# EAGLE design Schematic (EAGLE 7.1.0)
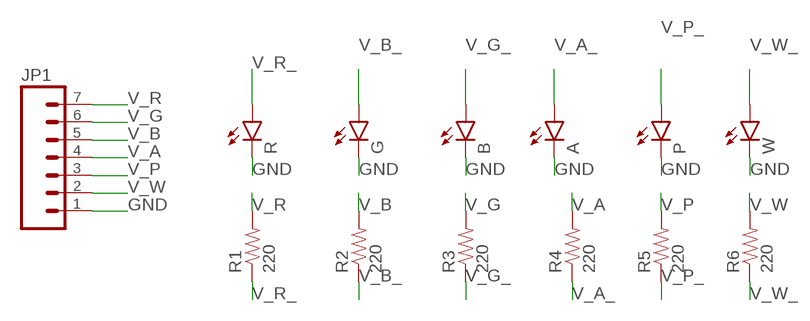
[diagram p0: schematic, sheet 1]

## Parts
A  LED5MM  [LED5MM]
B  LED5MM  [LED5MM]
G  LED5MM  [LED5MM]
JP1  M07  [1X07]
P  LED5MM  [LED5MM]
R  LED5MM  [LED5MM]
R1  220  RESISTOREZ  [AXIAL-0.3EZ]
R2  220  RESISTOREZ  [AXIAL-0.3EZ]
R3  220  RESISTOREZ  [AXIAL-0.3EZ]
R4  220  RESISTOREZ  [AXIAL-0.3EZ]
R5  220  RESISTOREZ  [AXIAL-0.3EZ]
R6  220  RESISTOREZ  [AXIAL-0.3EZ]
W  LED5MM  [LED5MM]

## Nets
GND: A.K(C) B.K(C) G.K(C) JP1.1 P.K(C) R.K(C) W.K(C)
V_A: JP1.4 R4.P$2
V_A_: A.A R4.P$1
V_B: JP1.5 R2.P$2
V_B_: G.A R2.P$1
V_G: JP1.6 R3.P$2
V_G_: B.A R3.P$1
V_P: JP1.3 R5.P$2
V_P_: P.A R5.P$1
V_R: JP1.7 R1.P$2
V_R_: R1.P$1 R.A
V_W: JP1.2 R6.P$2
V_W_: R6.P$1 W.A

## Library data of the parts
A B G P R W = SparkFun-LED:LED: LEDs
JP1 = SparkFun-Connectors:M07: Header 7 Standard 7-pin 0.1" header. Use with straight break away headers (SKU : PRT-00116), right angle break away headers (PRT-00553), swiss pins (PRT-00743), machine pins (PRT-00117), and female headers (PRT-00115). NOTES ON THE VARIANTS LOCK and LOCK_LONGPADS... This footprint was designed to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
R1-R6 = SparkFun-Passives:RESISTOR: Resistor

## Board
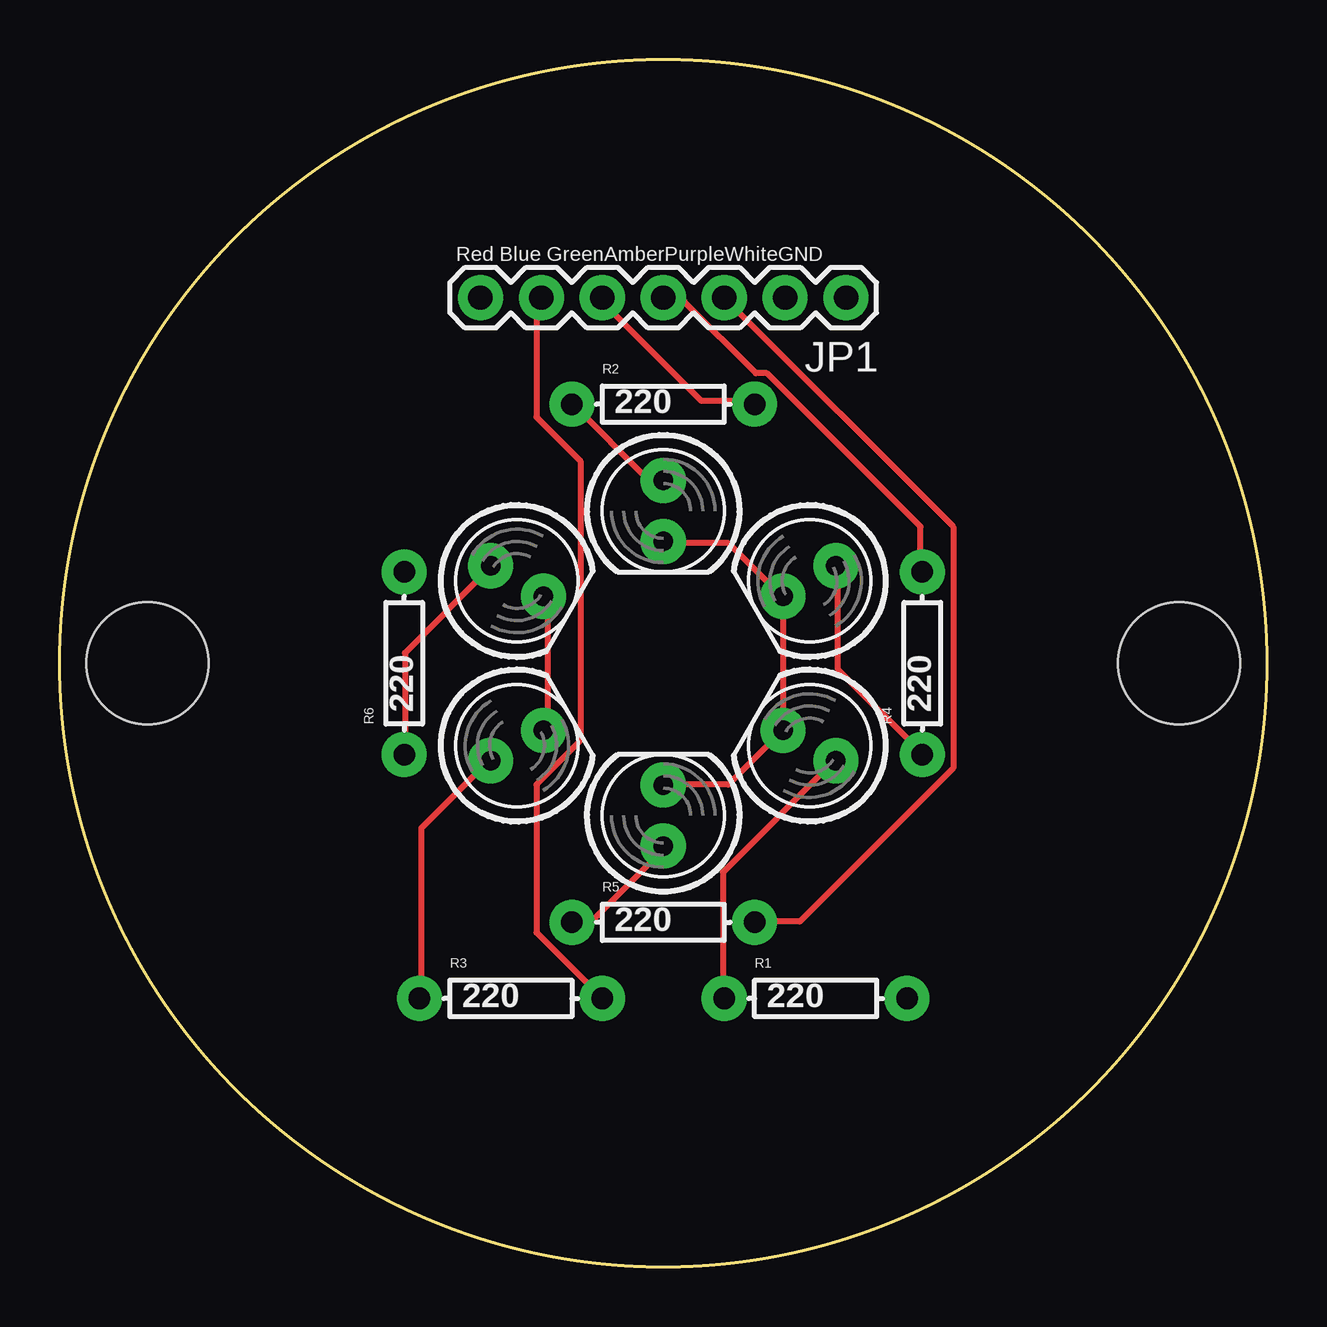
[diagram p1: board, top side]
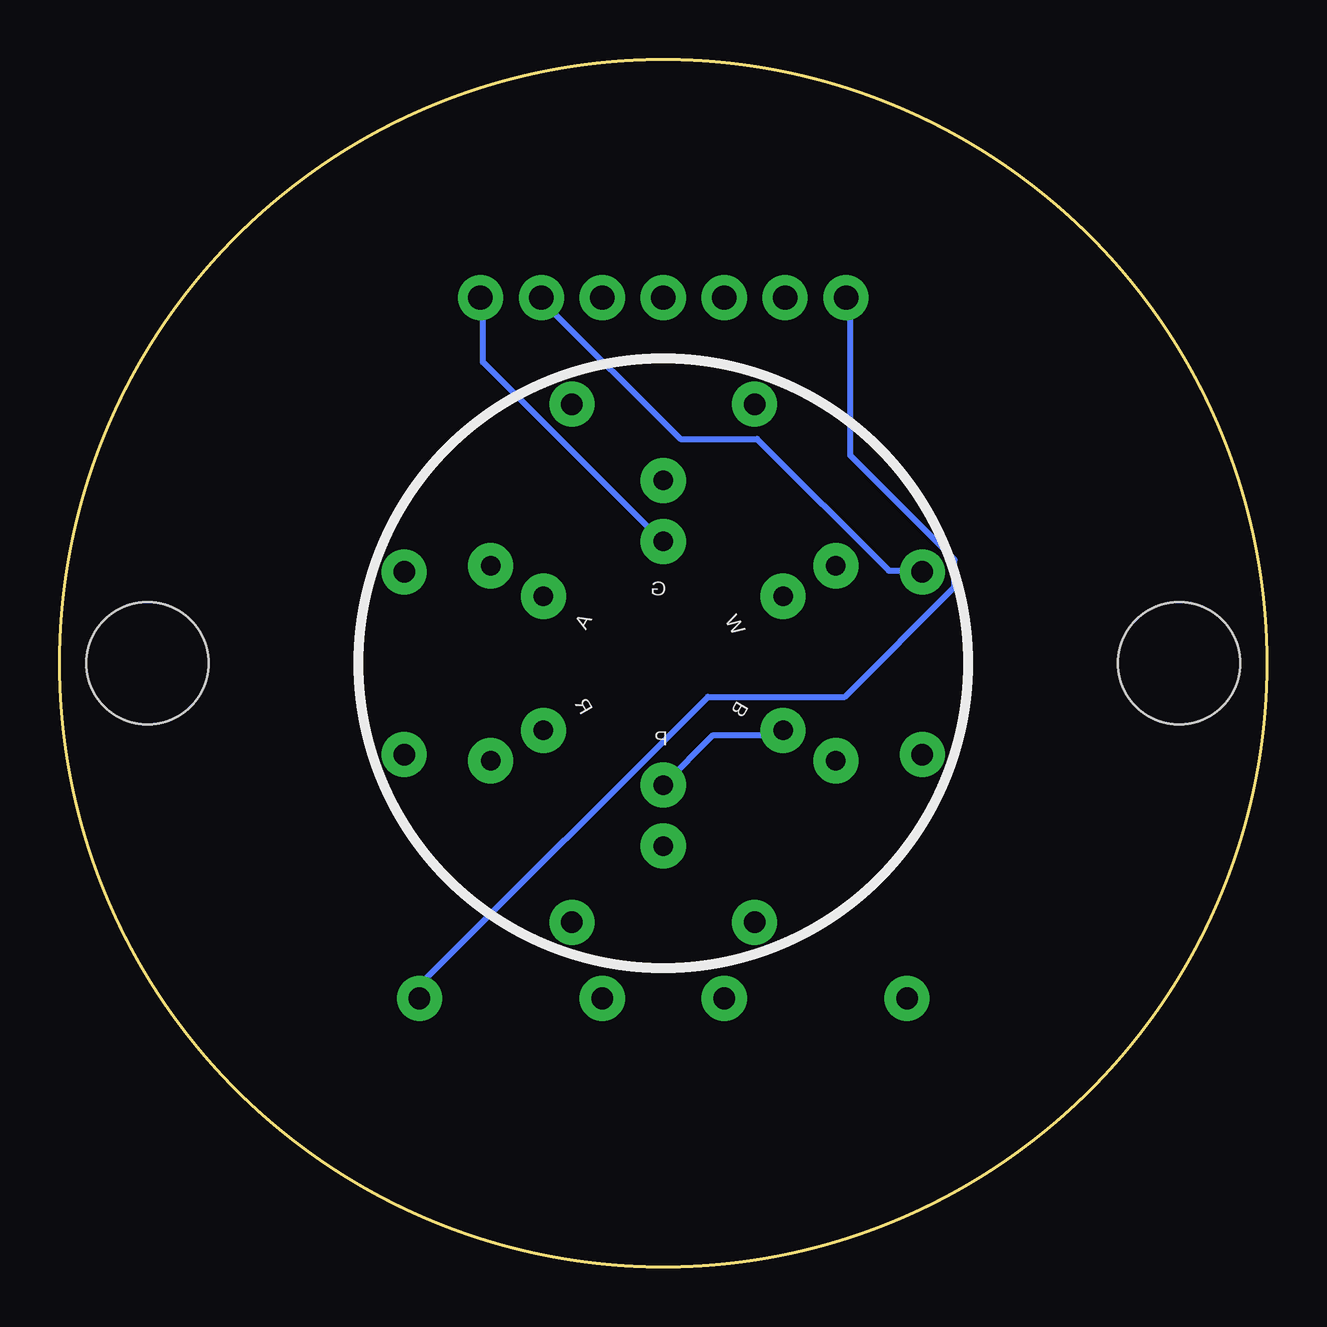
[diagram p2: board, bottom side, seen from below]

Size 50.29 x 50.29 mm. Coordinates in mm from the lower left corner, seen from the top.
Outline: circle at 25.15,25.15 radius 25.15
Copper layers (1*16): Top 0.035mm / dielectric 1.5mm / Bottom 0.035mm
Design rules "default": minimum track width 10mil, minimum drill 24mil, track to track 8mil, track to pad 8mil, pad to pad 8mil, via to via 8mil, smd to smd 8mil, copper to edge 40mil, drill to drill 8mil, minimum pad ring 10mil, minimum via ring 8mil, stop-mask expansion 4mil, vias tented up to drill 0mil, thermal gap 10mil
Holes 5.08 mm at 3.65,25.15 46.65,25.15

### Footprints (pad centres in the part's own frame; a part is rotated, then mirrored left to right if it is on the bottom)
LED5MM = drill 0.813 pad 1.88: A -1.27,0; K 1.27,0
1X07 = drill 1.016 pad 1.88: 1 0,0; 2 2.54,0; 3 5.08,0; 4 7.62,0; 5 10.16,0; 6 12.7,0; 7 15.24,0
AXIAL-0.3EZ = drill 0.9 pad 1.88: P$1 -3.81,0; P$2 3.81,0

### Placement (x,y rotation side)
A  31.24,28.58 210 top
B  19.05,21.72 30 top
G  25.15,31.5 270 top
JP1  32.77,40.39 180 top
P  25.15,18.8 90 top
R  31.24,21.72 150 top
R1  31.5,11.18 0 top
R2  25.15,35.94 0 top
R3  18.8,11.18 0 top
R4  35.94,25.15 90 top
R5  25.15,14.35 0 top
R6  14.35,25.15 90 top
W  19.05,28.58 330 top

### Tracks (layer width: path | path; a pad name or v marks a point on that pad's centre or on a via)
GND
  Top 0.254: B.K 20.32,22.38 20.32,27.86 W.K | P.K 25.35,20.09 27.86,20.09 29.92,22.15 R.K 30.15,22.38 30.15,27.86 A.K 29.92,28.09 27.86,30.15 25.35,30.15 G.K
  Bottom 0.254: JP1.1 32.66,40.21 32.66,37.69 25.35,30.38 G.K | P.K 23.06,22.15 20.32,22.15 B.K
V_A
  Top 0.254: JP1.4 25.35,40.21 26.04,40.21 29.01,37.24 29.46,37.24 35.87,30.84 35.87,29.01 R4.P$2
V_A_
  Top 0.254: A.A 32.44,29.01 32.44,24.89 35.87,21.46 R4.P$1
V_B
  Top 0.254: R2.P$2 28.78,36.09 26.72,36.09 22.61,40.21 JP1.5
V_B_
  Top 0.254: G.A 25.12,32.89 24.44,32.89 21.46,35.87 R2.P$1
V_G
  Top 0.254: R3.P$2 19.86,13.92 19.86,20.09 21.69,21.92 21.69,33.58 19.86,35.41 19.86,40.21 JP1.6
V_G_
  Top 0.254: R3.P$1 15.06,11.18 15.06,18.26 17.81,21.01 B.A
V_P
  Top 0.254: JP1.3 37.24,30.84 37.24,20.78 30.84,14.38 29.01,14.38 R5.P$2
V_P_
  Top 0.254: R5.P$1 21.46,14.38 22.15,14.38 25.12,17.35 P.A
V_R
  Bottom 0.254: JP1.7 17.35,40.21 17.35,33.81 13.01,29.46 13.01,28.32 17.58,23.75 23.29,23.75 35.18,11.86 35.18,11.18 R1.P$2
V_R_
  Top 0.254: R1.P$1 27.64,11.18 27.64,16.43 32.21,21.01 R.A
V_W
  Bottom 0.254: R6.P$2 14.38,29.01 15.75,29.01 21.23,34.49 24.44,34.49 30.15,40.21 JP1.2
V_W_
  Top 0.254: R6.P$1 14.38,21.46 14.38,25.58 17.81,29.01 W.A

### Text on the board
tPlace: Red Blue GreenAmberPurpleWhiteGND

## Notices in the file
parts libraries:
SparkFun-LED: Licensing: Creative Commons ShareAlike 4.0 International - https://creativecommons.org/licenses/by-sa/4.0
